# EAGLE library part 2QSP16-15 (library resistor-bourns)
BOURNS RESISTOR NETWORK
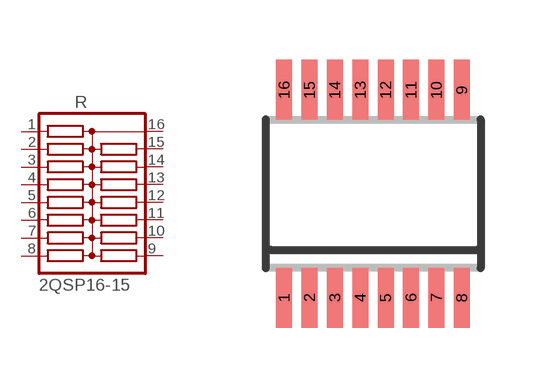
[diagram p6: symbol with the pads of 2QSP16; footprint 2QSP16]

Designator prefix R

## 2QSP16-15 (OC_FARNELL: unknown; OC_NEWARK: unknown)  [2QSP16]
1  1  pas
2  2  pas
3  3  pas
4  4  pas
5  5  pas
6  6  pas
7  7  pas
8  8  pas
9  9  pas
10  10  pas
11  11  pas
12  12  pas
13  13  pas
14  14  pas
15  15  pas
16  16  pas

## Footprint 2QSP16 (pad centres in mm)
BOURNS RESISTOR NETWORK
smd 0.4 x 1.5: 1 -2.223,-2.6; 2 -1.588,-2.6; 3 -0.953,-2.6; 4 -0.318,-2.6; 5 0.318,-2.6; 6 0.953,-2.6; 7 1.588,-2.6; 8 2.223,-2.6; 9 2.223,2.6; 10 1.588,2.6; 11 0.953,2.6; 12 0.318,2.6; 13 -0.318,2.6; 14 -0.953,2.6; 15 -1.588,2.6; 16 -2.223,2.6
